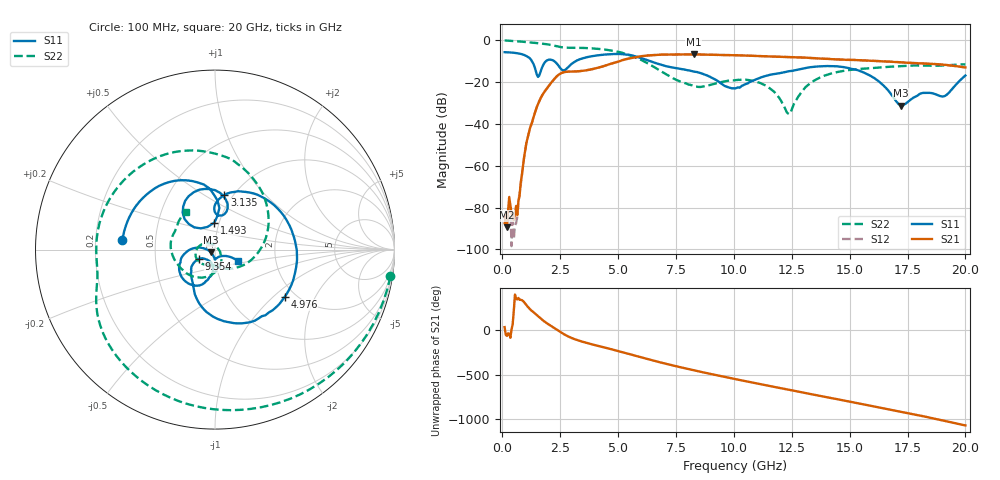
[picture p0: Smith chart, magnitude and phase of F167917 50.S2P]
!  2-Port S-parameters saved by WinCal
! VAR MeasName=S-Parameters (CALIBRATED_DATA) read from VNA (N5242A)
! VAR MeasDate=2016-11-22 9:02:21
! VAR NAME=F167917 50
! VAR FILENAME=F167917 50.S2P
! VAR DATE=2016-11-22 9:02:21
! VAR PHYS_PORTS=1,2
# Hz S DB R 50
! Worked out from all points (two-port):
!   401 points, 100 MHz to 20 GHz, reference 50 ohm
!   highest |S21| = -6.75 dB at 8.259 GHz (marker M1); lowest = -89.3 dB at 199.5 MHz (marker M2)
!   |S21| within 3 dB of the highest: 5.133 GHz to 15.85 GHz (10.72 GHz wide, 102 % of centre)
!   lowest |S11| = -31.2 dB at 17.21 GHz (marker M3), VSWR 1.06, Z = 47.8 - j1.53 ohm
!   |S11| at or under -10 dB: 1.279 GHz to 1.884 GHz (605.5 MHz wide, 38.3 % of centre); 2.246 GHz to 3.168 GHz (922.6 MHz wide, 34.1 % of centre); 6.388 GHz to end of sweep
!   |S22| runs from -35.3 to -0.1 dB; largest |S21 - S12| = 0.004
!   S11 on the Smith chart (normalised r, x): 100 MHz: 0.32, +0.05; 1.493 GHz: 0.95, +0.29; 3.135 GHz: 0.91, +0.61; 4.976 GHz: 1.76, -1.19; 9.354 GHz: 0.83, -0.09; 20 GHz: 1.28, -0.17
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1e8  -5.71 174.2  -87.49 32.8  -85.65 20.8  -0.10 -8.7
1.995e8  -5.74 168.3  -89.33 -66.2  -82.51 -9.1  -0.16 -16.9
6.4725e8  -6.21 141.1  -83.60 -15.2  -84.41 -43.2  -0.49 -52.2
1.04525e9  -7.56 112.7  -48.88 -81.6  -48.87 -81.3  -0.87 -80.8
1.493e9  -16.44 91.3  -31.81 167.8  -31.81 168.1  -1.35 -109.7
2.33875e9  -10.96 77.5  -17.43 6.6  -17.41 6.6  -2.81 -156.1
3.13475e9  -10.23 80.3  -14.92 -104.0  -14.92 -103.9  -3.59 175.3
3.43325e9  -8.77 61.9  -14.67 -129.5  -14.66 -129.6  -3.64 162.9
4.9755e9  -6.57 -34.1  -10.35 126.0  -10.33 126.2  -5.46 89.4
5.82125e9  -7.90 -82.8  -7.99 65.7  -7.96 65.8  -8.53 39.0
6.7665e9  -11.43 -115.1  -6.90 -0.1  -6.88 -0.0  -14.18 -22.1
8.259e9  -14.92 -137.6  -6.75 -91.7  -6.73 -91.6  -21.77 -99.0
9.3535e9  -19.83 -150.1  -7.05 -153.1  -7.05 -153.1  -20.25 -119.5
1.005e10  -23.02 -119.3  -7.16 169.3  -7.17 169.4  -19.13 -143.4
1.1443e10  -16.88 -98.1  -7.75 96.2  -7.68 96.4  -22.07 158.1
1.238825e10  -14.78 -105.8  -8.08 47.9  -8.04 47.8  -35.33 31.1
1.338325e10  -12.80 -119.1  -8.52 -3.6  -8.47 -3.6  -19.91 -77.5
1.507475e10  -13.67 -159.0  -9.38 -87.8  -9.35 -88.2  -14.11 -132.1
1.67165e10  -24.70 174.2  -10.19 -172.5  -10.25 -172.3  -12.68 -165.6
1.7214e10  -31.21 -144.5  -10.54 161.7  -10.53 161.6  -12.35 -175.3
1.91045e10  -26.67 -57.0  -11.76 58.8  -11.72 58.8  -12.09 148.0
2e10  -16.87 -26.4  -12.99 7.4  -12.92 7.6  -11.53 127.2
